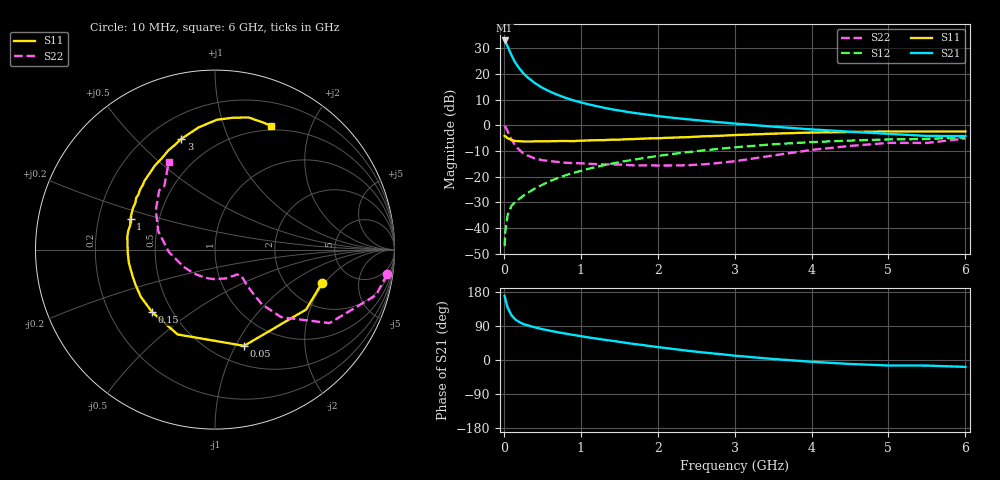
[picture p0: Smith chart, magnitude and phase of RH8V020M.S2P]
! SIEMENS Small Signal Semiconductors
! BFR106
! Si NPN RF Bipolar Junction Transistor in SOT23
! VCE = 8 V  IC = 20 mA
! Common Emitter S-Parameters:  August  1996
# GHz  S  MA  R  50
!  f  S11  S21  S12  S22
! GHz  MAG  ANG  MAG  ANG  MAG  ANG  MAG  ANG
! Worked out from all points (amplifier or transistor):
!   36 points, 10 MHz to 6 GHz, reference 50 ohm
!   highest |S21| = 33.1 dB at 10 MHz (marker M1)
!   |S21| within 3 dB of that: start of sweep to 58.91 MHz
!   unconditionally stable (mu >= 1): 380 MHz to 2.085 GHz
!   at 250 MHz: K = 0.88, MSG = 24.0 dB, |S12| = -27.5 dB
!   at 1.4 GHz: K = 1.06, MAG = 9.1 dB, |S12| = -15.0 dB
!   at 6 GHz: K = 0.99, MSG = 0.3 dB, |S12| = -4.7 dB
!   S11 on the Smith chart (normalised r, x): 10 MHz: 3.10, -1.87; 50 MHz: 0.69, -1.08; 150 MHz: 0.39, -0.36; 1 GHz: 0.34, +0.16; 3 GHz: 0.33, +0.69; 6 GHz: 0.45, +1.46
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0.01  0.6241 -17.2  45.13 169.0  0.0044 83.5  0.969 -8.1
0.02  0.6079 -33.3  42.95 160.1  0.0086 78.0  0.9327 -15.8
0.05  0.5602 -73.2  34.27 137.8  0.0181 61.5  0.7581 -32.7
0.1  0.5166 -113.8  23.11 117.8  0.0268 54.4  0.5271 -45.6
0.15  0.494 -135.1  16.6 106.7  0.0325 54.3  0.4016 -49.4
0.2  0.4899 -147.4  12.95 100.2  0.0366 56.3  0.3333 -49.1
0.25  0.4842 -155.7  10.49 95.3  0.042 57.8  0.2867 -48.5
0.3  0.4825 -162.1  8.825 92.0  0.0472 60.5  0.2611 -47.9
0.4  0.4857 -171.4  6.717 86.4  0.0581 63.6  0.227 -46.0
0.5  0.4866 -178.1  5.4 81.5  0.0693 65.4  0.2092 -44.9
0.6  0.4885 176.3  4.538 77.2  0.0817 65.9  0.2003 -45.5
0.7  0.4934 171.7  3.92 73.3  0.0934 66.9  0.1933 -46.8
0.8  0.4946 167.9  3.446 69.7  0.1059 66.5  0.1864 -48.1
1  0.5013 159.8  2.796 62.9  0.1293 66.1  0.1816 -52.3
1.1  0.5068 156.4  2.566 59.6  0.1418 65.6  0.1781 -55.7
1.6  0.5353 141.1  1.827 44.9  0.2028 61.2  0.1685 -73.5
2.2  0.5758 125.5  1.398 29.2  0.2768 54.3  0.1649 -103.0
3  0.645 106.9  1.082 11.4  0.3717 43.2  0.1993 -151.3
3.5  0.6869 97.6  0.942 2.7  0.4264 35.7  0.2574 -177.0
4.5  0.7413 82.3  0.75 -10.5  0.5037 19.9  0.396 146.4
5.5  0.7571 69.5  0.621 -14.7  0.5412 8.9  0.4532 128.5
6  0.7572 65.5  0.617 -18.2  0.581 1.2  0.5537 117.7
